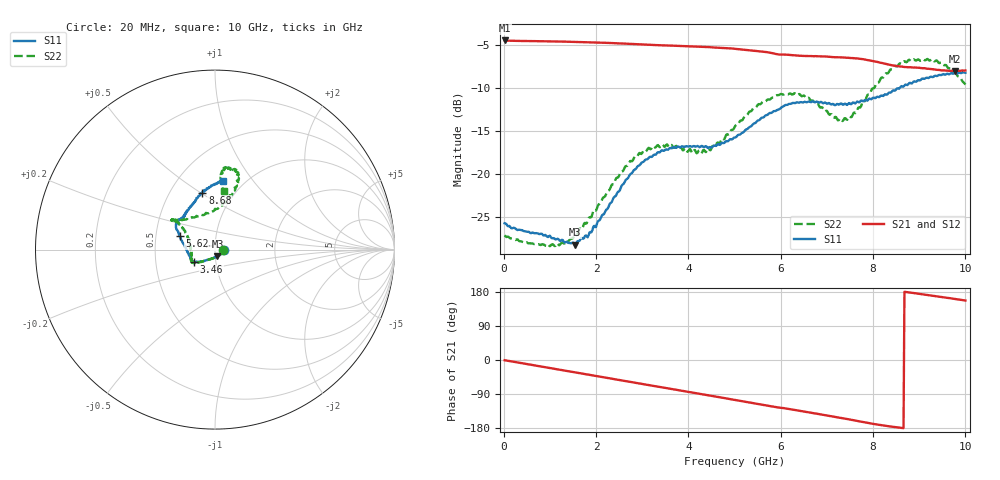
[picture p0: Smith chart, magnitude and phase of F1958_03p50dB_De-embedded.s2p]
! Integrated Device Technology
! Corporate Headquarters
! 6024 Silver Creek Valley Road
! San Jose, CA 95138  USA
! Phone:  1-408-284-8200
! Toll Free:  1-800-223-1366
! Webpage:  http://www.idt.com/
! Timing and RF Division
! 515 Groton Road, Suite 102
! Westford, MA 01886-6024
! Device:  F1958
! Description: 7-bit 0.25 dB Digital Step Attenuator
! Frequency:  0.001 -  6.000 GHz
! Package:  4x4 mm Thin QFN Plastic Package: 24 pin
! Ports:  2 RF, 12 DC
!  Pin  1  = D0
!  Pin  2  = VDD
!  Pin  3  = VMODE
!  Pin  4  = GND
!  Pin  5  = RF1  =  Port 1
!  Pin  6  = GND
!  Pin  7  = GND
!  Pin  8  = GND
!  Pin  9  = GND
!  Pin 10  = GND
!  Pin 11  = GND
!  Pin 12  = GND
!  Pin 13  = GND
!  Pin 14  = RF2  =  Port 2
!  Pin 15  = GND
!  Pin 16  = LE
!  Pin 17  = CLK
!  Pin 18  = DATA
!  Pin 19  = D6
!  Pin 20  = D5
!  Pin 21  = D4
!  Pin 22  = D3
!  Pin 23  = D2
!  Pin 24  = D1
! State:  14
! Atten State:  3.50 dB
! Voltage:  +3.30 Volts
! Current:  0.257 mA
! Data:  The device was measured on a F1958 evaluation board which has
!  individual transmission lines to the RF pins.  Data was collected
!  using a calibrated network analyzer.  The evaluation board was
!  de-embedded using Automatic Fixture Removal (AFR).
!  The reference plane is the edge of the package pin.
! Misc:
!  Action Tracker AT0419
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# GHz S dB R 50
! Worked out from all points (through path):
!   500 points, 20 MHz to 10 GHz, reference 50 ohm
!   highest |S21| = -4.52 dB at 20 MHz (marker M1); lowest = -8.1 dB at 9.78 GHz (marker M2)
!   group delay of S21, straight-line fit = 57.2 ps
!   lowest |S11| = -28.2 dB at 1.54 GHz (marker M3), VSWR 1.08, Z = 51.3 - j3.74 ohm
!   |S11| at or under -10 dB: start of sweep to 8.583 GHz
!   |S22| runs from -28.4 to -6.7 dB; largest |S21 - S12| = 0.0017
!   S11 on the Smith chart (normalised r, x): 20 MHz: 1.11, -0.00; 3.46 GHz: 0.78, -0.11; 5.62 GHz: 0.66, +0.11; 8.68 GHz: 0.72, +0.51; 10 GHz: 0.80, +0.72
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0.02  -25.72 -2.5  -4.52 -0.6  -4.52 -0.5  -27.12 -3.1
0.96  -27.32 -30.9  -4.62 -20.3  -4.62 -20.3  -28.15 -44.4
1.54  -28.20 -69.3  -4.69 -32.5  -4.68 -32.5  -27.08 -89.6
1.7  -27.43 -81.6  -4.71 -35.8  -4.71 -35.8  -26.38 -101.8
1.86  -26.78 -95.3  -4.73 -39.2  -4.72 -39.2  -25.03 -110.0
2.72  -20.20 -138.0  -4.91 -57.3  -4.89 -57.3  -18.68 -142.7
3.36  -17.50 -148.0  -5.07 -70.7  -5.07 -70.8  -16.77 -150.1
3.46  -17.32 -149.1  -5.09 -72.8  -5.09 -72.9  -16.70 -151.6
4.34  -16.89 -161.1  -5.26 -91.2  -5.28 -91.2  -17.21 178.7
5.02  -15.77 177.4  -5.49 -105.7  -5.50 -105.7  -14.39 150.0
5.62  -13.47 158.7  -5.82 -118.5  -5.83 -118.5  -11.59 144.1
6.18  -11.88 148.9  -6.19 -129.4  -6.21 -129.4  -10.71 145.2
6.68  -11.61 142.5  -6.34 -139.4  -6.35 -139.3  -11.50 141.1
7.2  -11.95 136.4  -6.47 -150.5  -6.48 -150.4  -13.41 118.6
7.4  -11.85 134.0  -6.51 -155.0  -6.52 -154.9  -13.53 103.7
7.6  -11.80 130.9  -6.59 -159.4  -6.59 -159.3  -12.88 89.9
7.92  -11.26 122.4  -6.82 -166.7  -6.82 -166.8  -10.78 76.3
8.34  -10.59 111.7  -7.31 -174.9  -7.32 -175.0  -8.20 71.0
8.68  -9.75 102.4  -7.59 180.0  -7.59 -180.0  -6.92 74.0
9.28  -8.77 89.9  -7.85 169.4  -7.86 169.4  -6.69 82.9
9.78  -8.27 84.5  -8.06 161.2  -8.08 161.2  -8.21 84.6
10  -8.27 83.8  -7.99 157.0  -8.02 157.1  -9.64 81.4
